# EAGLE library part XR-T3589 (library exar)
V.35/BELL 306 DRIVER/RECEIVER
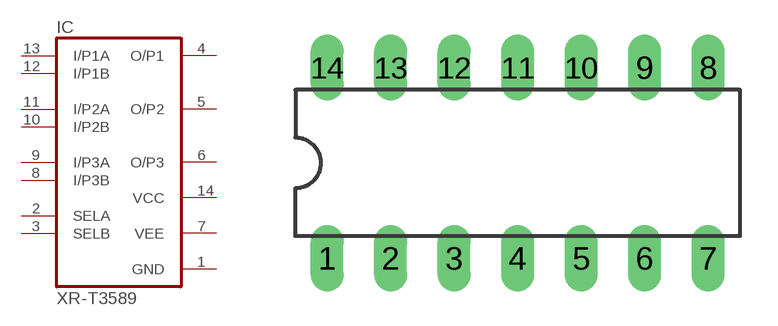
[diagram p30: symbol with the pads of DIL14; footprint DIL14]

Designator prefix IC

## XR-T3589 (OC_FARNELL: unknown; OC_NEWARK: unknown)  [DIL14]
1  GND  pwr
2  SELA  in
3  SELB  in
4  O/P1  out
5  O/P2  out
6  O/P3  out
7  VEE  pwr
8  I/P3B  in
9  I/P3A  in
10  I/P2B  in
11  I/P2A  in
12  I/P1B  in
13  I/P1A  in
14  VCC  pwr

## Footprint DIL14 (pad centres in mm)
Dual In Line Package
drill 0.813 long: 1 -7.62,-3.81; 2 -5.08,-3.81; 3 -2.54,-3.81; 4 0,-3.81; 5 2.54,-3.81; 6 5.08,-3.81; 7 7.62,-3.81; 8 7.62,3.81; 9 5.08,3.81; 10 2.54,3.81; 11 0,3.81; 12 -2.54,3.81; 13 -5.08,3.81; 14 -7.62,3.81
